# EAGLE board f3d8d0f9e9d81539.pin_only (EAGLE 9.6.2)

Size 15.49 x 27.94 mm. Coordinates in mm from the lower left corner, seen from the top.
Outline: 15.49,1.27 15.49,26.67 arc90 14.22,27.94 1.27,27.94 arc90 0,26.67 0,1.27 arc90 1.27,0 14.22,0 arc90 15.49,1.27
Copper layers (1*16): Top 0.035mm / dielectric 1.5mm / Bottom 0.035mm
Design rules "default": minimum track width 8mil, minimum drill 0.4mm, track to track 8mil, track to pad 8mil, pad to pad 8mil, via to via 8mil, smd to smd 8mil, copper to edge 20mil, drill to drill 8mil, minimum pad ring 8mil, minimum via ring 10mil, stop-mask expansion 3mil, vias tented up to drill 0mil, thermal gap 8mil

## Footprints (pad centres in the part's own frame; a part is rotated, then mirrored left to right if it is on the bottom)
C0805 = smd 1.3 x 1.5: 1 -0.85,0; 2 0.85,0
1X10_ROUND_76 = drill 1 pad 1.93: 1 -11.43,0; 2 -8.89,0; 3 -6.35,0; 4 -3.81,0; 5 -1.27,0; 6 1.27,0; 7 3.81,0; 8 6.35,0; 9 8.89,0; 10 11.43,0
R0805 = smd 1.1 x 1.4: 1 -1,0; 2 1,0
TSSOP20 = smd 0.305 x 0.991: 1 -2.925,-2.918; 2 -2.275,-2.918; 3 -1.625,-2.918; 4 -0.975,-2.918; 5 -0.325,-2.918; 6 0.325,-2.918; 7 0.975,-2.918; 8 1.625,-2.918; 9 2.275,-2.918; 10 2.925,-2.918; 11 2.925,2.918; 12 2.275,2.918; 13 1.625,2.918; 14 0.975,2.918; 15 0.325,2.918; 16 -0.325,2.918; 17 -0.975,2.918; 18 -1.625,2.918; 19 -2.275,2.918; 20 -2.925,2.918
FIDUCIAL_1MM = smd 1 x 1: 1 0,0

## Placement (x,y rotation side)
C1  0.1uF  [C0805]  6.22,21.59 270 top
C2  0.1uF  [C0805]  9.02,21.59 270 top
JP1  [1X10_ROUND_76]  14.1,13.72 270 top
JP2  [1X10_ROUND_76]  1.4,13.72 90 top
R1  10K  [R0805]  7.62,3.05 0 top
U1  TXB0108PWR  [TSSOP20]  7.75,13.72 270 top
U$4  [ADAFRUIT200MIL]  7.37,18.67 270 top
U$6  FIDUCIAL  [FIDUCIAL_1MM]  7.75,13.72 0 top

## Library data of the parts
C1 C2 R1 U$4 U$6 = adafruit
JP1 JP2 U1 = microbuilder

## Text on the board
tPlace: 1.2-3.6V | 1.7-5.5V | VCCB | VCCA | B1 | A1 | B2 | A2 | B3 | A3 | B4 | A4 | B5 | A5 | B6 | A6 | TXB0108 | Level | B7 | A7 | Shifter | B8 | A8 | GND | OE | Bidirectional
